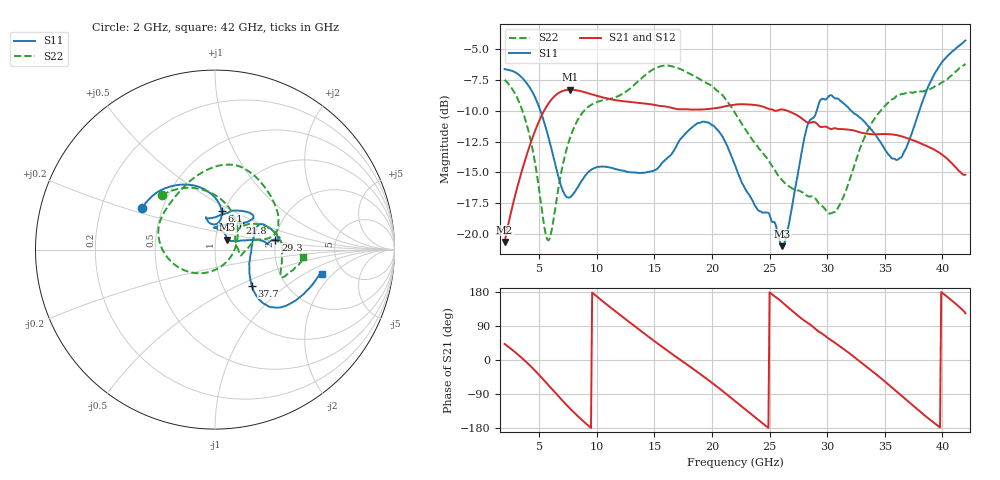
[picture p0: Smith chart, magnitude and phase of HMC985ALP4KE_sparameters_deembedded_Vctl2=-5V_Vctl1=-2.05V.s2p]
!s2p File: Measurements: S11, S21, S12, S22
# GHz S dB R 50.0
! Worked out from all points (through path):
!   401 points, 2 GHz to 42 GHz, reference 50 ohm
!   highest |S21| = -8.27 dB at 7.7 GHz (marker M1); lowest = -20.7 dB at 2 GHz (marker M2)
!   lowest |S11| = -21.0 dB at 26.1 GHz (marker M3), VSWR 1.20, Z = 57.1 + j6.4 ohm
!   |S11| at or under -10 dB: 5.113 GHz to 29.09 GHz (23.98 GHz wide, 140 % of centre); 32.1 GHz to 37.99 GHz (5.89 GHz wide, 16.8 % of centre)
!   |S22| runs from -20.6 to -6.2 dB; largest |S21 - S12| = 0.00048
!   S11 on the Smith chart (normalised r, x): 2 GHz: 0.39, +0.23; 6.1 GHz: 0.98, +0.44; 21.8 GHz: 1.26, +0.38; 29.3 GHz: 1.99, +0.25; 37.7 GHz: 1.36, -0.60; 42 GHz: 3.46, -1.50
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2  -6.60 150.0  -20.68 42.3  -20.68 42.3  -7.46 134.3
3.3  -7.11 129.3  -15.54 10.7  -15.54 10.7  -9.38 101.3
4.5  -8.62 106.9  -11.99 -23.7  -11.99 -23.7  -13.49 59.5
5.6  -11.45 86.4  -9.70 -59.5  -9.71 -59.5  -20.17 -20.0
6.1  -13.22 80.4  -9.04 -76.5  -9.04 -76.5  -19.66 -77.6
7.7  -17.03 94.3  -8.28 -128.8  -8.28 -128.8  -12.14 -162.4
8.7  -15.68 104.3  -8.42 -157.9  -8.42 -157.9  -10.22 173.7
12.2  -14.86 105.1  -9.21 114.8  -9.21 114.8  -8.63 126.4
15.4  -14.57 85.3  -9.59 40.8  -9.60 40.9  -6.42 82.1
18.4  -11.25 50.2  -9.90 -24.3  -9.90 -24.3  -7.15 48.8
21.8  -13.94 46.7  -9.52 -103.5  -9.52 -103.4  -9.86 12.6
22  -14.42 49.4  -9.49 -108.4  -9.50 -108.4  -10.16 12.0
24.1  -18.16 90.0  -9.58 -159.9  -9.58 -159.8  -13.09 12.4
26.1  -21.02 38.8  -9.88 152.3  -9.89 152.4  -15.65 -3.7
28.7  -10.62 5.6  -10.92 89.5  -10.92 89.5  -16.95 -9.1
29.3  -9.35 9.4  -11.24 74.5  -11.24 74.5  -17.57 -4.2
30.8  -8.98 13.3  -11.44 42.6  -11.45 42.6  -18.15 25.6
32.4  -10.25 26.5  -11.63 6.5  -11.63 6.6  -14.34 40.8
35.4  -13.63 7.0  -11.90 -66.9  -11.90 -66.8  -9.27 16.6
37.7  -10.85 -44.4  -12.48 -126.8  -12.47 -126.7  -8.47 -6.5
39.8  -6.26 -41.4  -13.45 -178.2  -13.45 -178.2  -7.77 -22.0
42  -4.27 -12.8  -15.20 123.3  -15.20 123.4  -6.16 -4.6
